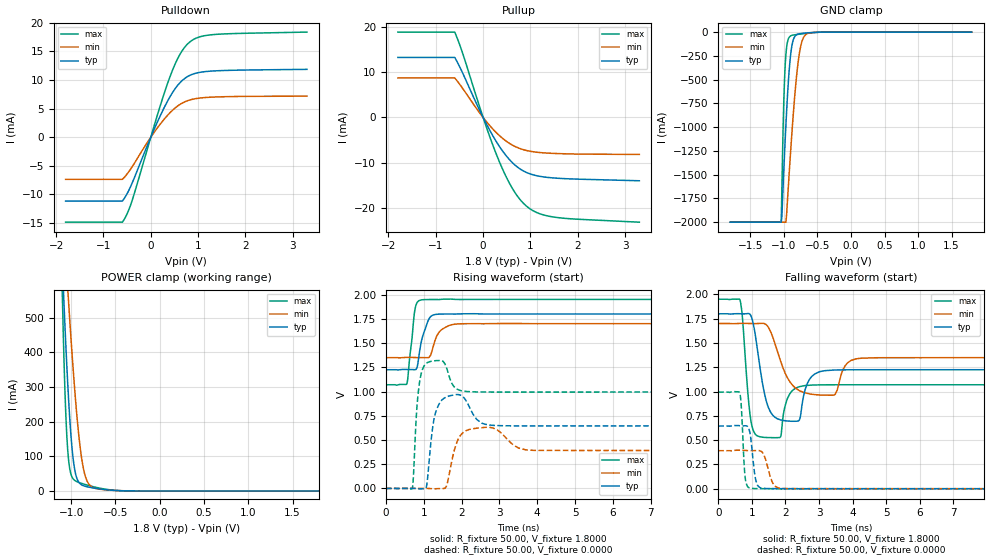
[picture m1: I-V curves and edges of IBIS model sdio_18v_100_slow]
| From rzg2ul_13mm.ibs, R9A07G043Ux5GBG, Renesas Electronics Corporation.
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[Model]   sdio_18v_100_slow
Model_type   I/O
Polarity   Non-Inverting
Enable   Active-Low
Vinl  =   0.5800V
Vinh  =   1.2700V
Vmeas =   0.9000V
Cref  =   10.00pF
| variable   typ   min   max
C_comp   3.085e-12  2.97e-12  3.085e-12
[Model Spec]
| Subparameter   typ   min   max
| Thresholds
Vinh   0.5800   NA   NA
Vinl   1.2700   NA   NA
| Timing Thresholds
Vmeas   0.9000   0.8500   0.9750
| variable   typ   min   max
[Temperature Range]   25.000   125.000   -40.000
| variable   typ   min   max
[Voltage Range]   1.800V   1.700V   1.950V
| variable   typ   min   max
[Pullup Reference]   1.800V   1.700V   1.950V
| variable   typ   min   max
[Pulldown Reference]   0.000V   0.000V   0.000V
| variable   typ   min   max
[POWER Clamp Reference] 1.800V   1.700V   1.950V
| variable   typ   min   max
[GND Clamp Reference]   0.000V   0.000V   0.000V
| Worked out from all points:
|   slope of the pulldown table from 0 to 0.27 V, typ, clamps not added: 54.5 ohm
|   slope of the pullup table from 0 to 0.27 V, typ, clamps not added: 52.2 ohm
|   GND clamp passes 1 mA (typ) near -0.46 V on its own axis
|   POWER clamp passes 1 mA (typ) near -0.48 V on its own axis
|   rising waveform, R_fixture 50.00, V_fixture 1.8000: 20-80 % time 210ps typ, 227ps min, 139ps max; typ from 1.22 V to 1.8 V
|   rising waveform, R_fixture 50.00, V_fixture 0.0000: 20-80 % time 92.8ps typ, 121ps min, 75.4ps max; typ from 0 V to 0.645 V
|   falling waveform, R_fixture 50.00, V_fixture 1.8000: 20-80 % time 155ps typ, 216ps min, 108ps max; typ from 1.8 V to 1.22 V
|   falling waveform, R_fixture 50.00, V_fixture 0.0000: 20-80 % time 125ps typ, 199ps min, 85.1ps max; typ from 0.645 V to 0 V
[Pulldown]
| sdio_18v_100_slow Pulldown S28FDSIO_IBIS
| Wed Sep  2 14:14:58 2020
| voltage   I(typ)   I(min)   I(max)
-1.8V     -11.16mA   -7.359mA   -14.84mA
-600mV    -11.16mA   -7.359mA   -14.84mA
-500mV    -9.853mA   -6.416mA   -13.36mA
-400mV    -8.125mA   -5.246mA   -11.19mA
90mV      1.733mA    1.069mA    2.518mA
270mV     4.951mA    3.012mA    7.318mA
410mV     7.129mA    4.306mA    10.67mA
620mV     9.543mA    5.738mA    14.52mA
830mV     10.82mA    6.511mA    16.67mA
1.03V     11.31mA    6.83mA     17.51mA
1.34V     11.57mA    7.012mA    17.93mA
3.3V      11.85mA    7.17mA     18.35mA
[Pullup]
| sdio_18v_100_slow Pullup S28FDSIO_IBIS
| Wed Sep  2 14:14:58 2020
| voltage   I(typ)   I(min)   I(max)
-1.8V     13.25mA    8.73mA     18.84mA
-600mV    13.25mA    8.73mA     18.84mA
-430mV    9.747mA    6.375mA    14.07mA
20mV      -418.5uA   -268.2uA   -624.1uA
340mV     -6.326mA   -3.954mA   -9.686mA
490mV     -8.481mA   -5.239mA   -13.16mA
640mV     -10.18mA   -6.218mA   -16.03mA
790mV     -11.42mA   -6.902mA   -18.23mA
940mV     -12.24mA   -7.34mA    -19.76mA
1.19V     -12.97mA   -7.725mA   -21.21mA
1.54V     -13.38mA   -7.948mA   -22.04mA
3.3V      -13.96mA   -8.158mA   -23.1mA
[GND Clamp]
| sdio_18v_100_slow GNDClamp S28FDSIO_IBIS
| Wed Sep  2 14:14:58 2020
| voltage   I(typ)   I(min)   I(max)
-1.8V     -2A        -2A        -2A
-1.04V    -2A        -2A        -2A
-1.03V    -1.932A    -2A        -1.644A
-1.01V    -1.591A    -2A        -948.5mA
-990mV    -1.27A     -2A        -485.9mA
-960mV    -836.4mA   -1.924A    -160.7mA
-910mV    -308.8mA   -1.364A    -45.24mA
-860mV    -81.11mA   -862.2mA   -30.85mA
-790mV    -20.98mA   -328.8mA   -23.83mA
-740mV    -14.08mA   -121mA     -19.54mA
-670mV    -9.363mA   -24.28mA   -13.84mA
1.8V      0A         0A         0A
[POWER Clamp]
| sdio_18v_100_slow PWRClamp S28FDSIO_IBIS
| Wed Sep  2 14:14:58 2020
| voltage   I(typ)   I(min)   I(max)
-1.8V     2A         2A         2A
-1.1V     651.8mA    840.5mA    559.9mA
-1.09V    589.6mA    796.8mA    454.6mA
-1.06V    415.3mA    668.7mA    212.9mA
-1.03V    265.3mA    545.8mA    89.35mA
-1V       149.8mA    429.9mA    45.65mA
-970mV    76.02mA    323.1mA    32.36mA
-920mV    27.24mA    174mA      25.09mA
-880mV    17.2mA     90.23mA    21.57mA
-810mV    11.45mA    23.27mA    16.22mA
-670mV    5.368mA    4.716mA    7.629mA
1.8V      0A         0A         0A
[Ramp]
dV/dt_r   0.387/92.828p   0.235/120.831p  0.597/75.387p
dV/dt_f   0.345/153.462p  0.210/215.308p  0.528/107.305p
R_load = 50.00ohm
[Rising Waveform]
| sdio_18v_100_slow Rising-High S28FDSIO_IBIS
| Wed Sep  2 14:14:58 2020
R_fixture = 50.00
V_fixture = 1.8000
V_fixture_min = 1.7000
V_fixture_max = 1.9500
C_fixture = 0.00pF
| Time   V(typ)   V(min)   V(max)
0s        1.224V     1.349V     1.07V
550ps     1.228V     1.352V     1.077V
580ps     1.227V     1.352V     1.136V
770ps     1.225V     1.351V     1.848V
830ps     1.256V     1.35V      1.92V
930ps     1.5V       1.35V      1.945V
1.19ns    1.775V     1.381V     1.949V
1.42ns    1.798V     1.618V     1.949V
1.81ns    1.799V     1.694V     1.951V
10ns      1.8V       1.7V       1.95V
[Rising Waveform]
| sdio_18v_100_slow Rising-Low S28FDSIO_IBIS
| Wed Sep  2 14:14:58 2020
R_fixture = 50.00
V_fixture = 0.0000
C_fixture = 0.00pF
| Time   V(typ)   V(min)   V(max)
0s        0V         0V         0V
700ps     200uV      500uV      1.9mV
890ps     -5.4mV     100uV      1.093V
1.07ns    16.5mV     100uV      1.29V
1.17ns    393mV      -1.6mV     1.309V
1.53ns    928.4mV    -900uV     1.303V
1.92ns    967.9mV    514.4mV    1.017V
2.4ns     712.7mV    621.3mV    995.6mV
3.71ns    645mV      396.9mV    994.3mV
10ns      645mV      391.2mV    994.5mV
[Falling Waveform]
| sdio_18v_100_slow Falling-High S28FDSIO_IBIS
| Wed Sep  2 14:14:58 2020
R_fixture = 50.00
V_fixture = 1.8000
V_fixture_min = 1.7000
V_fixture_max = 1.9500
C_fixture = 0.00pF
| Time   V(typ)   V(min)   V(max)
0s        1.8V       1.7V       1.95V
650ps     1.801V     1.701V     1.94V
980ps     1.775V     1.7V       684.4mV
1.26ns    1.207V     1.701V     533mV
1.85ns    708.6mV    1.32V      532mV
2.19ns    694mV      1.075V     1.004V
2.87ns    1.181V     968.6mV    1.067V
3.48ns    1.222V     970.4mV    1.07V
4.1ns     1.224V     1.336V     1.07V
10ns      1.224V     1.349V     1.07V
[Falling Waveform]
| sdio_18v_100_slow Falling-Low S28FDSIO_IBIS
| Wed Sep  2 14:14:58 2020
R_fixture = 50.00
V_fixture = 0.0000
C_fixture = 0.00pF
| Time   V(typ)   V(min)   V(max)
0s        645mV      391.2mV    994.5mV
640ps     648.2mV    396.2mV    985.2mV
690ps     647mV      395.9mV    830.3mV
800ps     647.7mV    394.1mV    123.8mV
950ps     561.9mV    391.3mV    5.9mV
1.12ns    86.1mV     392.7mV    1.4mV
1.31ns    4.733mV    375.9mV    600uV
1.61ns    880uV      67.1mV     300uV
1.89ns    475uV      3.271mV    -4.686mV
10ns      0V         0V         0V
